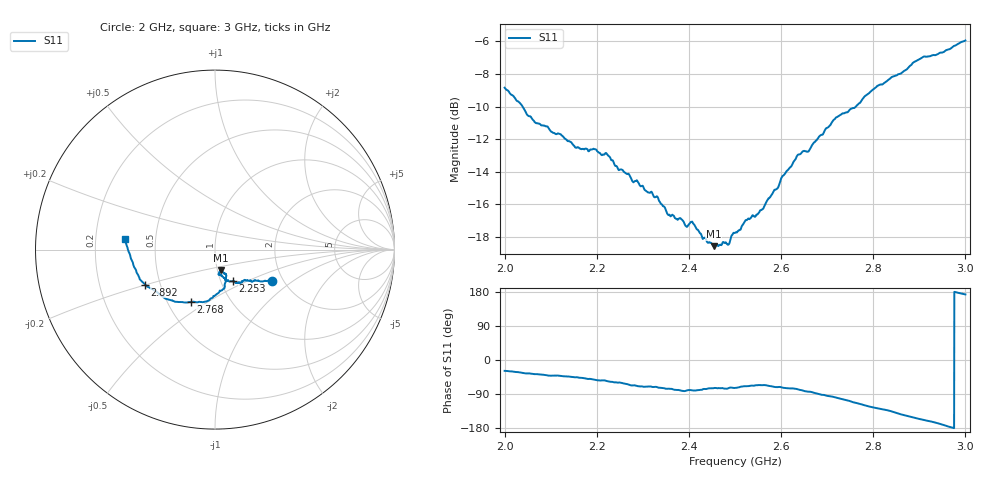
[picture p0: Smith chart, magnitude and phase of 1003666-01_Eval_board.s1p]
# Hz S DB R 50
! Planar, Obzor-804, 15045142, 19.1.3/3
! Date: 2/14/2023 4:30:46 PM
! Data: Format (Calibration Info)
! Freq	S11:dB/Ang(F1)
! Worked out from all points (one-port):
!   2001 points, 2 GHz to 3 GHz, reference 50 ohm
!   lowest |S11| = -18.6 dB at 2.454 GHz (marker M1), VSWR 1.27, Z = 51.9 - j12 ohm
!   |S11| at or under -10 dB: 2.039 GHz to 2.762 GHz (723.6 MHz wide, 30.1 % of centre)
!   S11 on the Smith chart (normalised r, x): 2 GHz: 1.75, -0.70; 2.253 GHz: 1.14, -0.42; 2.768 GHz: 0.65, -0.42; 2.892 GHz: 0.41, -0.20; 3 GHz: 0.33, +0.05
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2e9  -8.85 -28.7
2.0655e9  -10.96 -37.2
2.125e9  -11.79 -42.5
2.155e9  -12.53 -45.5
2.2225e9  -12.92 -55.7
2.25e9  -13.87 -59.5
2.2535e9  -13.86 -60.4
2.2925e9  -14.79 -69.8
2.332e9  -15.55 -72.2
2.3565e9  -16.65 -75.6
2.375e9  -16.94 -79.2
2.395e9  -17.37 -80.7
2.408e9  -17.11 -80.5
2.429e9  -18.06 -78.2
2.4535e9  -18.56 -74.2
2.485e9  -18.46 -74.8
2.5e9  -17.74 -73.7
2.5605e9  -16.27 -66.4
2.625e9  -13.50 -75.0
2.667e9  -12.38 -84.8
2.7165e9  -10.77 -98.2
2.75e9  -10.17 -108.7
2.7675e9  -9.85 -114.8
2.8335e9  -8.35 -133.5
2.875e9  -7.66 -148.1
2.8915e9  -7.23 -153.4
2.939e9  -6.80 -166.4
3e9  -5.95 173.0
